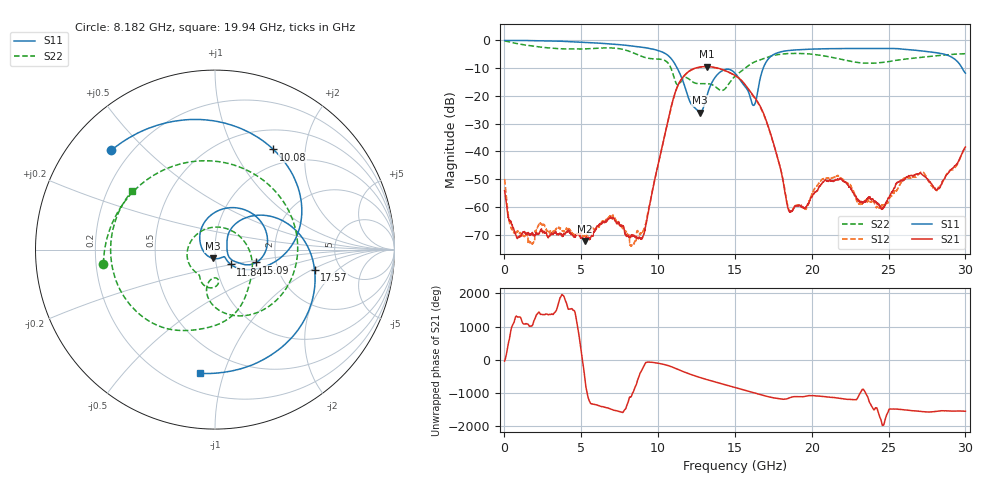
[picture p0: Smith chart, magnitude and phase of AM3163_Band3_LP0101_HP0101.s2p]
!Agilent Technologies,E8364B,MY43040894,A.07.50.67
!Agilent E8364B: A.07.50.67
!Date: Thursday, August 20, 2020 11:06:05
!Correction: S11(Full 2 Port(1,2))
!S21(Full 2 Port(1,2))
!S12(Full 2 Port(1,2))
!S22(Full 2 Port(1,2))
!S2P File: Measurements: S11, S21, S12, S22:
# Hz S  dB  R 50
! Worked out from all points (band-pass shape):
!   3201 points, 10 MHz to 30 GHz, reference 50 ohm
!   highest |S21| = -9.44 dB at 13.16 GHz (marker M1); lowest = -72.3 dB at 5.24 GHz (marker M2)
!   |S21| within 3 dB of the highest: 11.74 GHz to 14.95 GHz (3.203 GHz wide, 24 % of centre)
!   lowest |S11| = -26.0 dB at 12.73 GHz (marker M3), VSWR 1.11, Z = 48.6 - j4.75 ohm
!   |S11| at or under -10 dB: 11.24 GHz to 16.84 GHz (5.6 GHz wide, 39.9 % of centre); 29.79 GHz to end of sweep
!   |S22| runs from -18.1 to -0.2 dB; largest |S21 - S12| = 0.0048
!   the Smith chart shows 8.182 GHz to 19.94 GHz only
!   S11 on the Smith chart (normalised r, x): 8.182 GHz: 0.13, +0.40; 10.08 GHz: 0.76, +1.46; 11.84 GHz: 1.17, -0.20; 15.09 GHz: 1.58, -0.24; 17.57 GHz: 3.22, -1.08; 19.94 GHz: 0.31, -0.83
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1e7  -0.04 -1.9  -54.15 -41.2  -49.95 -52.5  -0.23 -6.4
1.040906e9  -0.05 -28.4  -70.65 -159.4  -69.55 77.6  -1.39 -85.1
2.352969e9  -0.13 -64.1  -68.28 -72.9  -66.00 -19.8  -2.44 -168.2
5.014581e9  -0.65 -134.4  -70.98 172.3  -70.14 30.1  -3.11 50.5
5.239506e9  -0.72 -140.3  -72.28 127.6  -70.80 42.5  -3.07 37.9
7.038906e9  -1.35 170.8  -64.06 -71.5  -63.00 -72.5  -2.74 -77.8
8.182275e9  -1.94 136.2  -70.93 -44.5  -73.60 -10.1  -4.06 -172.9
1.000979e10  -3.68 63.2  -44.39 -107.0  -44.56 -108.2  -6.74 -2.7
1.007539e10  -3.80 59.7  -42.74 -112.3  -42.91 -114.3  -6.77 -9.6
1.183731e10  -18.38 -43.2  -11.93 -35.9  -12.01 -35.6  -13.41 -102.0
1.272763e10  -26.00 -103.4  -9.62 -177.8  -9.67 -177.4  -15.61 -126.6
1.315874e10  -20.25 149.8  -9.44 121.6  -9.51 121.8  -15.60 -142.9
1.5005e10  -11.81 -12.6  -12.63 -116.5  -12.67 -116.4  -12.94 -22.7
1.508935e10  -12.37 -17.2  -12.93 -127.6  -12.96 -127.5  -12.53 -28.9
1.623272e10  -23.41 8.1  -20.19 84.0  -20.41 84.2  -7.89 -82.8
1.757289e10  -4.94 -11.5  -38.28 -76.1  -38.40 -73.0  -5.36 -131.3
1.855694e10  -3.63 -55.4  -61.83 -70.9  -61.36 -70.7  -4.74 -166.1
1.994398e10  -3.17 -97.1  -56.60 -4.0  -56.28 -6.1  -4.95 144.9
2.000958e10  -3.15 -98.9  -56.46 -6.6  -55.18 3.6  -4.99 142.5
2.274617e10  -2.92 -162.7  -55.35 -126.9  -54.68 -168.6  -7.77 20.1
2.500479e10  -3.00 144.9  -56.75 -88.0  -57.80 -56.9  -7.68 -91.8
3e10  -11.82 -21.9  -38.44 -116.2  -38.79 -116.0  -4.80 103.0
